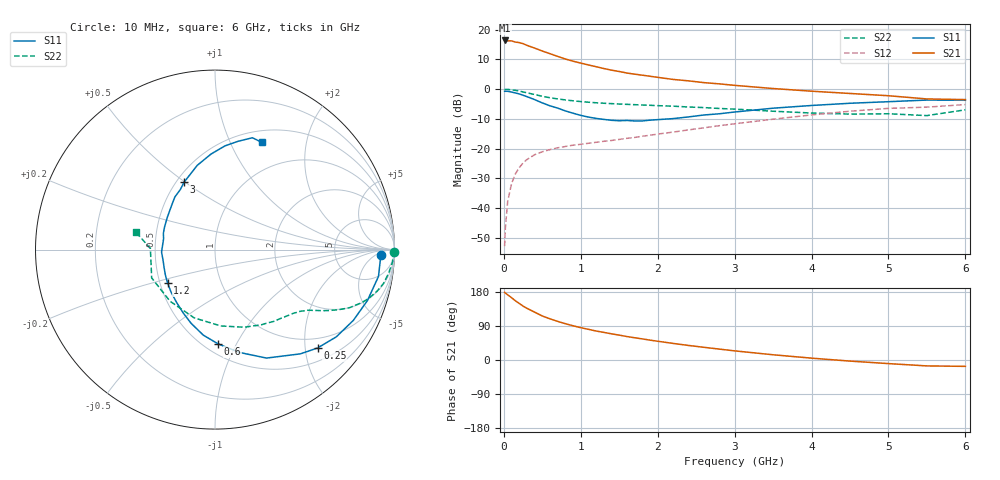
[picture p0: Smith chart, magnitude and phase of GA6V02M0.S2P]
! Infineon Technologies  Discrete & RF Semiconductors
! BF775
! Si NPN RF Bipolar Junction Transistor in SOT23
! VCE = 6 V  IC = 2 mA
! Common Emitter S-Parameters:  May  1996
# GHz  S  MA  R  50
!  f  S11  S21  S12  S22
! GHz  MAG  ANG  MAG  ANG  MAG  ANG  MAG  ANG
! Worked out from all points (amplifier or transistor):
!   36 points, 10 MHz to 6 GHz, reference 50 ohm
!   highest |S21| = 16.4 dB at 10 MHz (marker M1)
!   |S21| within 3 dB of that: start of sweep to 444.2 MHz
!   unconditionally stable (mu >= 1): 1.2 GHz to 3.389 GHz
!   at 250 MHz: K = 0.28, MSG = 20.1 dB, |S12| = -24.8 dB
!   at 1.4 GHz: K = 1.09, MAG = 10.0 dB, |S12| = -17.2 dB
!   at 6 GHz: K = 0.96, MSG = 0.8 dB, |S12| = -5.2 dB
!   S11 on the Smith chart (normalised r, x): 10 MHz: 21, -9; 250 MHz: 0.77, -2.26; 600 MHz: 0.58, -0.85; 1.2 GHz: 0.55, -0.23; 3 GHz: 0.55, +0.50; 6 GHz: 0.64, +1.33
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0.01  0.9233 -1.9  6.599 178.6  0.0023 87.4  0.9982 -0.7
0.02  0.923 -3.4  6.494 176.6  0.0047 85.7  0.9907 -1.5
0.05  0.9231 -9.3  6.505 172.1  0.013 84.6  0.992 -3.9
0.1  0.8954 -18.5  6.489 164.5  0.0258 79.1  0.9761 -7.8
0.15  0.8657 -27.1  6.198 156.3  0.0377 74.4  0.9577 -11.4
0.2  0.8326 -35.7  6.076 149.3  0.0481 69.7  0.9319 -14.4
0.25  0.7919 -43.8  5.832 142.3  0.0575 65.5  0.8997 -17.5
0.3  0.7507 -50.7  5.461 136.4  0.0657 62.8  0.8705 -19.8
0.4  0.669 -64.6  4.913 126.3  0.0793 56.6  0.8145 -23.5
0.5  0.5886 -76.7  4.384 116.2  0.0888 52.6  0.7604 -26.2
0.6  0.5256 -88.1  3.951 108.6  0.0966 49.9  0.7184 -28.2
0.8  0.4315 -108.0  3.218 95.8  0.109 46.9  0.6604 -30.9
0.9  0.3948 -116.7  2.955 90.3  0.1147 46.4  0.6387 -32.0
1.1  0.3401 -136.2  2.559 80.9  0.1235 46.4  0.6046 -34.3
1.2  0.3231 -144.9  2.386 76.5  0.1282 46.5  0.5914 -35.4
1.6  0.2981 -177.3  1.869 61.9  0.1495 48.1  0.5567 -40.3
2.2  0.3205 146.1  1.461 43.8  0.1901 50.1  0.5187 -50.3
3  0.4136 114.5  1.161 24.1  0.2623 48.2  0.4628 -69.2
3.5  0.4797 101.9  1.027 13.8  0.3134 44.4  0.4265 -85.7
4.5  0.5806 84.5  0.848 -2.9  0.4267 32.8  0.3815 -131.0
5.5  0.6571 71.5  0.686 -15.6  0.4995 16.4  0.3601 179.0
6  0.6518 66.3  0.669 -16.8  0.5522 11.9  0.4505 167.6
